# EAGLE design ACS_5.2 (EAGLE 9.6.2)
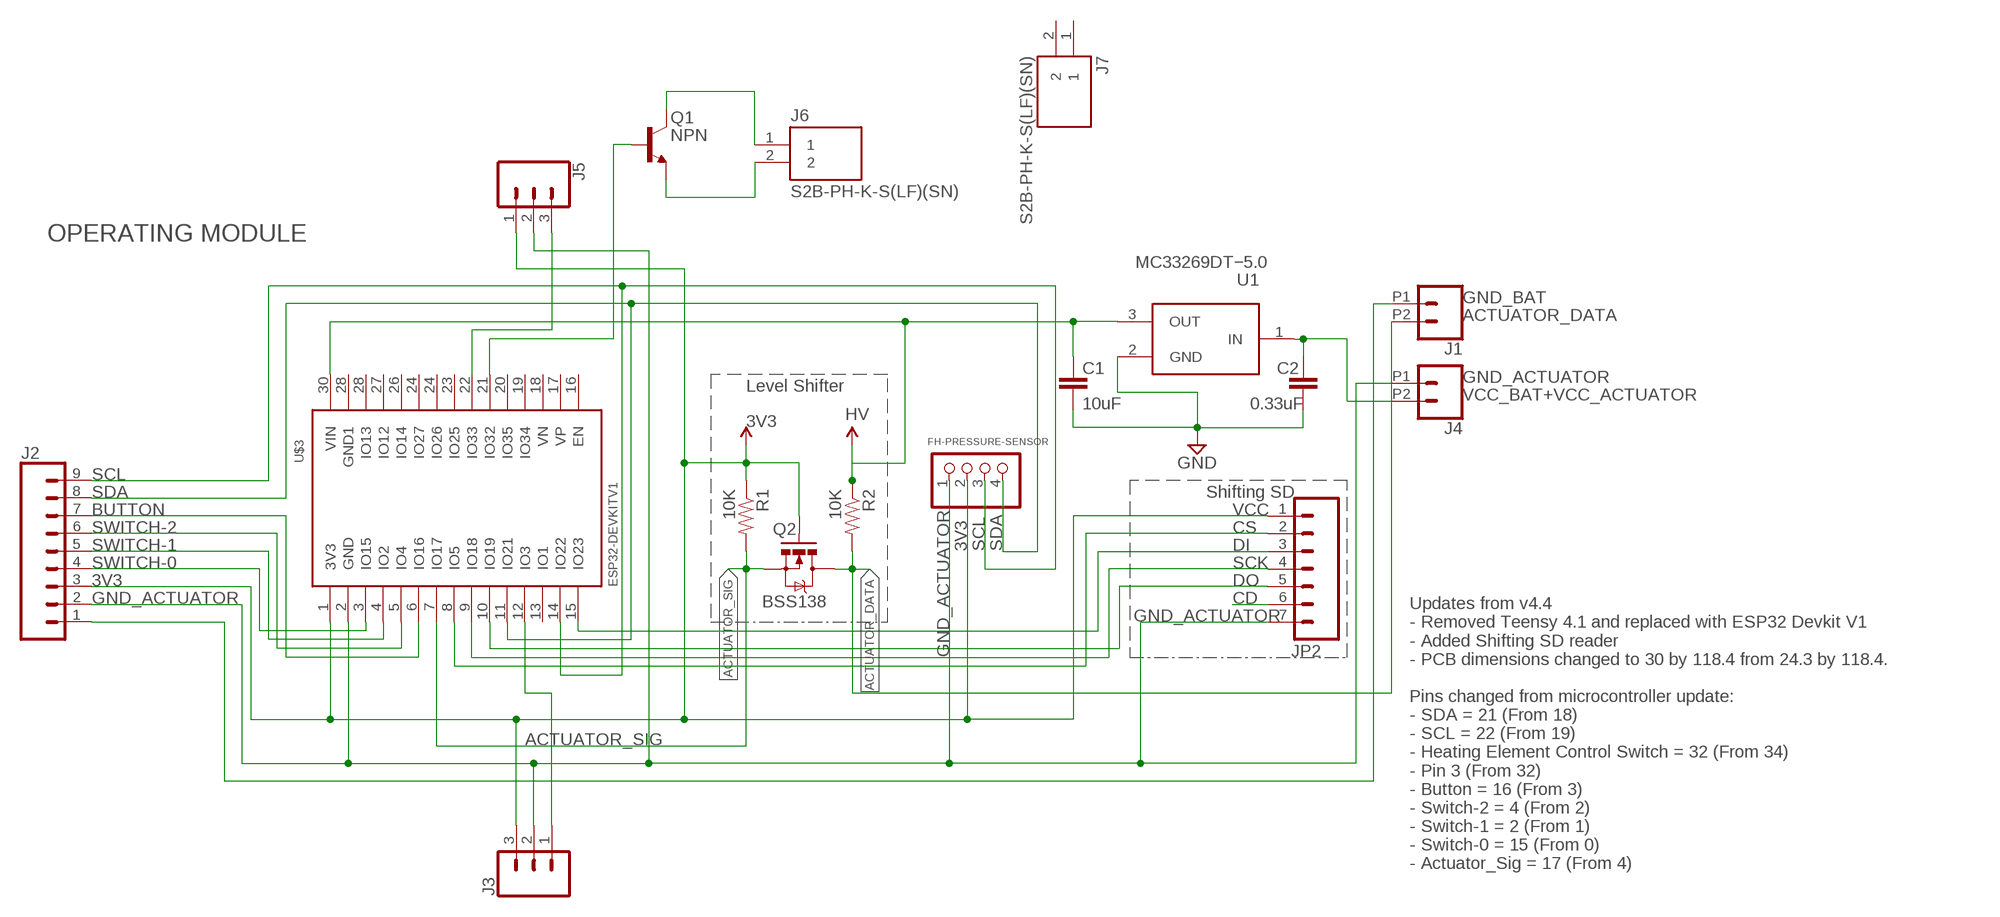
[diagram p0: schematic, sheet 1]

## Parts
C1  10uF  C_CHIP-0603(1608-METRIC)  [CAPC1608X85]
C2  0.33uF  C_CHIP-0603(1608-METRIC)  [CAPC1608X85]
FH-PRESSURE-SENSOR  PINHD-1X4  [1X04]
J1  CONN_022.54MM_SCREWTERM  [1X02_2.54_SCREWTERM]
J2  CONN_09  [1X09]
J3  CONN_03  [1X03]
J4  CONN_022.54MM_SCREWTERM  [1X02_2.54_SCREWTERM]
J5  CONN_03  [1X03]
J6  S2B-PH-K-S(LF)(SN)  [JST_S2B-PH-K-S(LF)(SN)]
J7  S2B-PH-K-S(LF)(SN)  [JST_S2B-PH-K-S(LF)(SN)]
JP2  M07  [1X07]
Q1  NPN  NPN_SOT23  [SOT95P237X112-3N]
Q2  BSS138  MOSFET-NCHANNELSMD  [SOT23-3]
R1  10K  RESISTOR0603-RES  [0603-RES]
R2  10K  RESISTOR0603-RES  [0603-RES]
U1  MC78M05BDTRKG  [MC78M05BDTRKG]
U$3  ESP32DEVKITV1  [ESP32-DEVKITV1]

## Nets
3V3: FH-PRESSURE-SENSOR.2 J2.3 J3.3 J5.1 JP2.1 Q2.1(G) R1.1 U$3.1(3V3) ; supply symbol labelled LV
ACTUATOR_DATA: J1.P2 Q2.3(D) R2.2
ACTUATOR_SIG: Q2.2(S) R1.2 U$3.7(IO17)
BUTTON: J2.7 U$3.6(IO16)
GND: C1.2 C2.2 U1.2(GND)
GND_ACTUATOR: FH-PRESSURE-SENSOR.1 J2.2 J3.2 J4.P1 J5.2 JP2.7 U$3.2(GND)
GND_BAT: J1.P1 J2.1
HV: C1.1 R2.1 U1.3(OUT) U$3.30(VIN)
N$1: J5.3 U$3.22(IO33)
N$3: J6.1 Q1.3(C)
N$4: J6.2 Q1.1(E)
N$5: Q1.2(B) U$3.21(IO32)
N$8: JP2.6
N$10: J3.1 U$3.12(IO3)
N$11: JP2.3 U$3.15(IO23)
N$12: JP2.2 U$3.8(IO5)
N$13: JP2.4 U$3.9(IO18)
N$14: JP2.5 U$3.10(IO19)
SCL: FH-PRESSURE-SENSOR.3 J2.9 U$3.14(IO22)
SDA: FH-PRESSURE-SENSOR.4 J2.8 U$3.11(IO21)
SWITCH-0: J2.4 U$3.3(IO15)
SWITCH-1: J2.5 U$3.4(IO2)
SWITCH-2: J2.6 U$3.5(IO4)
VCC_BAT+VCC_ACTUATOR: C2.1 J4.P2 U1.1(IN)
Unconnected: J7.1 J7.2 U$3.13(IO1) U$3.16(EN) U$3.17(VP) U$3.18(VN) U$3.19(IO34) U$3.20(IO35) U$3.23(IO25) U$3.24(IO26) U$3.24(IO27) U$3.26(IO14) U$3.27(IO12) U$3.28(GND1) U$3.28(IO13)

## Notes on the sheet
- Heating Element 
  Control Switch
- OPERATING MODULE
- Actuator Voltage: 7.5 MAX
- MC33269DT−5.0
- Level Shifter
- Shifting SD
- VCC
- CS
- DI
- SCK
- DO
- CD
- Updates from v4.4
  - Removed Teensy 4.1 and replaced with ESP32 Devkit V1
  - Added Shifting SD reader
  - PCB dimensions changed to 30 by 118.4 from 24.3 by 118.4.
  
  Pins changed from microcontroller update:
  - SDA = 21 (From 18)
  - SCL = 22 (From 19)
  - Heating Element Control Switch = 32 (From 34)
  - Pin 3 (From 32)
  - Button = 16 (From 3)
  - Switch-2 = 4 (From 2)
  - Switch-1 = 2 (From 1)
  - Switch-0 = 15 (From 0)
  - Actuator_Sig = 17 (From 4)

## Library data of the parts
C1 C2 = Capacitor:C: Capacitor - Generic; CATEGORY: Capacitor
FH-PRESSURE-SENSOR = pinhead:PINHD-1X4: PIN HEADER
J1 J4 = SparkFun-Connectors:CONN_02: Multi connection point. Often used as Generic Header-pin footprint for 0.1 inch spaced/style header connections
J2 = SparkFun-Connectors:CONN_09: Multi connection point. Often used as Generic Header-pin footprint for 0.1 inch spaced/style header connections On any of the 0.1 inch spaced packages, you can populate with these: Break Away Headers - Straight (PRT-00116) Break Away Male Headers - Right Angle (PRT-00553) Female Headers (PRT-00115)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
J3 J5 = SparkFun-Connectors:CONN_03: Multi connection point. Often used as Generic Header-pin footprint for 0.1 inch spaced/style header connections On any of the 0.1 inch spaced packages, you can populate with these: Break Away Headers - Straight (PRT-00116) Break Away Male Headers - Right Angle (PRT-00553) Female Headers (PRT-00115)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
J6 J7 = S2B-PH-K-S_LF__SN_:S2B-PH-K-S(LF)(SN): PH Series 2 Position 2.0 mm Through Hole Side Entry Shrouded Header Check availability; AVAILABILITY: In Stock; DESCRIPTION: Connector Header Through Hole, Right Angle 2 position; MF: JST Sales America Inc.; MP: S2B-PH-K-S(LF)(SN); PACKAGE: None; PRICE: None; PURCHASE-URL: https://pricing.snapeda.com/search/part/S2B-PH-K-S(LF)(SN)/?ref=eda
JP2 = SparkFun-Connectors:M07: Header 7 Standard 7-pin 0.1" header. Use with straight break away headers (SKU : PRT-00116), right angle break away headers (PRT-00553), swiss pins (PRT-00743), machine pins (PRT-00117), and female headers (PRT-00115). NOTES ON THE VARIANTS LOCK and LOCK_LONGPADS... This footprint was designed to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
Q1 = Transistor:NPN: NPN - Generic; CATEGORY: Transistor; SUB-CATEGORY: BJT; TYPE: NPN
Q2 = SparkFun:MOSFET-NCHANNEL
R1 R2 = SparkFun:RESISTOR: Resistor
U1 = LDO:MC78M05BDTRKG: IC REG LINEAR 5V 500MA DPAK Manufacturer's datasheet; CREATED_BY: PCBLayout.com; DIGIKEY_PN: MC78M05BDTRKGOSCT-ND; MANUFACTURER: ON Semiconductor; MPN: IC REG LINEAR 5V 500MA DPAK; PACKAGE: DPak
U$3 = ESP32-DEVKITV1:ESP32DEVKITV1

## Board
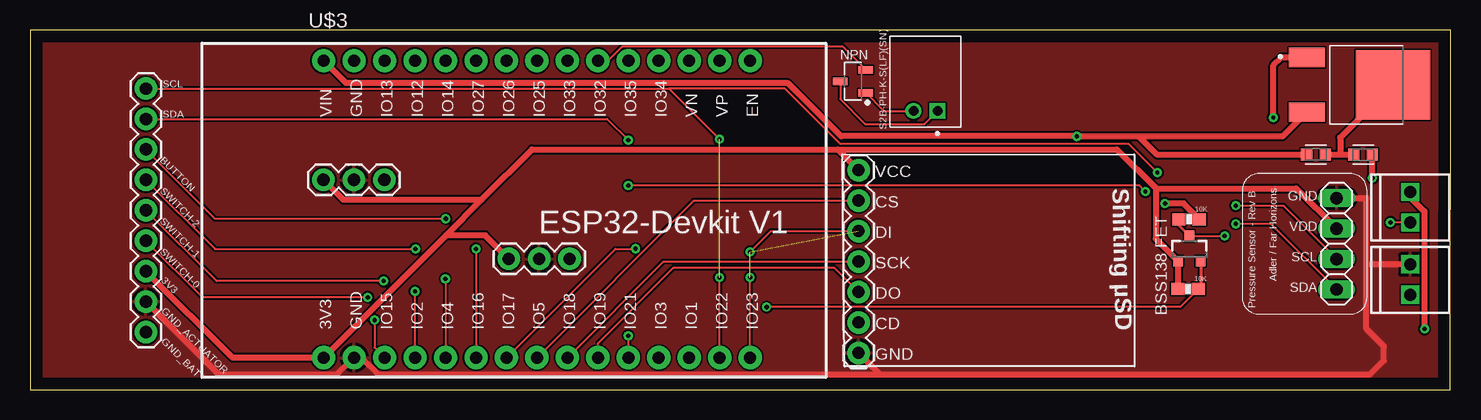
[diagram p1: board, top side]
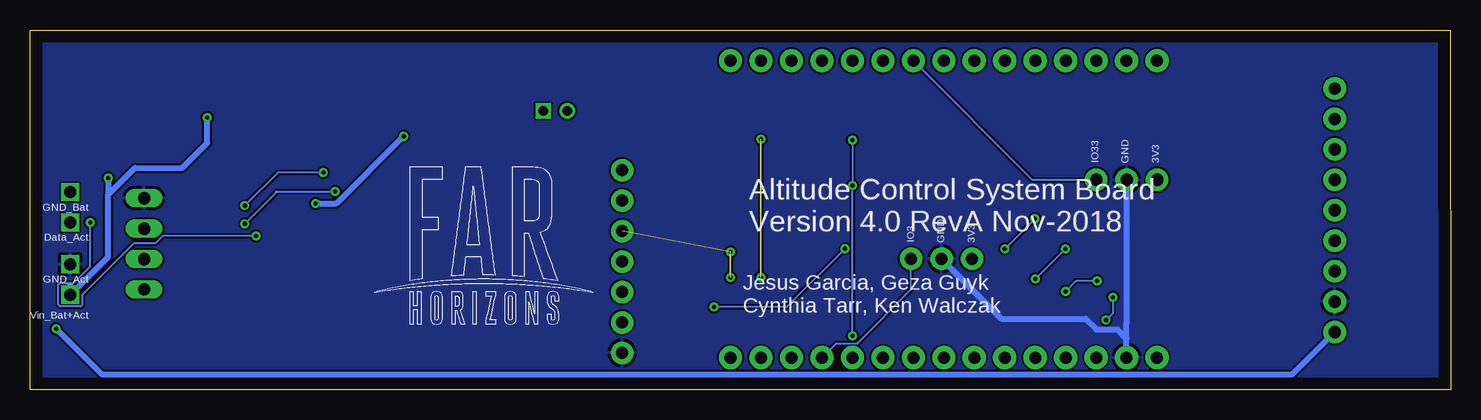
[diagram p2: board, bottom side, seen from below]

Size 118.43 x 30 mm. Coordinates in mm from the lower left corner, seen from the top.
Outline: 0,0 118.4,0 118.43,30 0.03,30 0,0
Copper layers (1*16): Top 0.035mm / dielectric 1.5mm / Bottom 0.035mm
Design rules "default": minimum track width 6mil, minimum drill 0.35mm, track to track 6mil, track to pad 6mil, pad to pad 6mil, via to via 6mil, smd to smd 6mil, copper to edge 40mil, drill to drill 6mil, minimum pad ring 10mil, minimum via ring 8mil, stop-mask expansion 4mil, vias tented up to drill 0mil, thermal gap 10mil

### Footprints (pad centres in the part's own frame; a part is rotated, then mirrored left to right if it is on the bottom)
CAPC1608X85 = smd 0.921 x 0.97: 1 -0.775,0; 2 0.775,0
1X04 = drill 1.016 long: 1 -3.81,0; 2 -1.27,0; 3 1.27,0; 4 3.81,0
1X02_2.54_SCREWTERM = drill 1.016 square: P1 2.54,0; P2 0,0
1X09 = drill 1.016 pad 1.88: 1 0,0; 2 2.54,0; 3 5.08,0; 4 7.62,0; 5 10.16,0; 6 12.7,0; 7 15.24,0; 8 17.78,0; 9 20.32,0
1X03 = drill 1.016 pad 1.88: 1 0,0; 2 2.54,0; 3 5.08,0
JST_S2B-PH-K-S(LF)(SN) = drill 0.8 square: 1 -1,0 | drill 0.8: 2 1,0
1X07 = drill 1.016 pad 1.88: 1 0,0; 2 2.54,0; 3 5.08,0; 4 7.62,0; 5 10.16,0; 6 12.7,0; 7 15.24,0
SOT95P237X112-3N = smd 1.224 x 0.625: 1 -1.064,0.95; 2 -1.064,-0.95; 3 1.064,0
SOT23-3 = smd 0.8 x 0.9: 1 -0.95,-1; 2 0.95,-1; 3 0,1.1
0603-RES = smd 1.1 x 1: 1 -0.85,0; 2 0.85,0
MC78M05BDTRKG = smd 1.6 x 3: 1 -2.285,-4.08; 3 2.285,-4.08 | smd 5.8 x 6.2: 2 0,3.1
ESP32-DEVKITV1 = drill 1 pad 1.93: 1 -22.87,-13.54; 2 -20.33,-13.54; 3 -17.79,-13.54; 4 -15.25,-13.54; 5 -12.71,-13.54; 6 -10.17,-13.54; 7 -7.63,-13.54; 8 -5.09,-13.54; 9 -2.55,-13.54; 10 -0.01,-13.54; 11 2.53,-13.54; 12 5.07,-13.54; 13 7.61,-13.54; 14 10.15,-13.54; 15 12.69,-13.54; 16 12.69,11.23; 17 10.15,11.23; 18 7.61,11.23; 19 5.07,11.23; 20 2.53,11.23; 21 -0.01,11.23; 22 -2.55,11.23; 23 -5.09,11.23; 24 -7.63,11.23; 25 -10.17,11.23; 26 -12.71,11.23; 27 -15.25,11.23; 28 -17.79,11.23; 29 -20.33,11.23; 30 -22.87,11.23

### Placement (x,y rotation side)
C1  107.19,19.61 0 top
C2  111.13,19.6 180 top
FH-PRESSURE-SENSOR  108.92,12.15 270 top
J1  115.07,13.94 90 top
J2  9.66,4.79 90 top
J3  44.98,10.9 180 top
J4  115.07,7.91 90 top
J5  24.46,17.5 0 top
J6  74.65,23.25 180 top
J7  not placed on the board
JP2  69.07,18.3 270 top
Q1  68.61,25.72 180 top
Q2  96.65,11.72 0 top
R1  96.56,8.41 0 top
R2  96.62,14.21 180 top
U1  110.51,25.42 270 top
U$3  47.34,16.2 0 top

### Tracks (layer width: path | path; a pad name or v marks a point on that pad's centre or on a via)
3V3
  Top 0.152: 95.7,8.42 R1.1
  Top 0.254: 95.68,10.73 Q2.1
  Top 0.508: J2.3 16.88,2.65 U$3.1 34.67,12.86 | 34.67,12.86 37.66,15.85 | 37.66,15.85 41.84,20.03 67.34,20.03 | JP2.1 67.34,20.03 | 67.34,20.03 90.6,20.03 93.84,16.79 93.84,16.78 | 93.84,16.78 105.56,16.78 FH-PRESSURE-SENSOR.2 | 93.84,16.78 93.84,12.57 Q2.1 95.69,10.71 95.69,8.42 R1.1 | J5.1 26.11,15.85 37.66,15.85 | J3.3 37.94,12.86 34.67,12.86
ACTUATOR_DATA  (via drill 0.35)
  Top 0.152: Q2.3 v99.59,12.82 | J1.P2 v113.41,13.94
  Top 0.254: R2.2 95.77,13.7 Q2.3
  Bottom 0.152: v99.59,12.82 107.36,12.82 107.98,12.2 109.76,12.2 114.08,7.89 114.08,7.05 114.21,6.92 115.93,6.92 116.06,7.05 116.06,8.76 115.93,8.9 114.77,8.9 113.41,10.26 v113.41,13.94
ACTUATOR_SIG  (via drill 0.35)
  Top 0.152: 97.47,8.48 R1.2 95.88,6.88 v61.41,6.88 | U$3.7 48.8,11.75 v50.48,11.75
  Top 0.254: Q2.2 97.6,8.6 97.47,8.48
  Bottom 0.152: v50.48,11.75 55.35,6.88 v61.41,6.88
BUTTON  (via drill 0.35)
  Top 0.152: v37.17,11.74 U$3.6 | v34.66,14.25 15.44,14.25 J2.7
  Bottom 0.152: v34.66,14.25 v37.17,11.74
GND
  Top 0.508: C1.2 109.22,19.61 | 109.22,19.61 110.34,19.61 C2.2 | 109.22,19.61 109.22,21.03 U1.2
GND_ACTUATOR
  Top 0.508: J2.2 15.73,1.27 25.62,1.27 U$3.2 27.61,2.67 29.01,1.27 70.86,1.27 | 70.86,1.27 111.7,1.27 112.86,2.43 112.86,3.6 111.4,5.06 111.4,10.61 | JP2.7 70.86,1.27 | J4.P1 111.56,10.45 111.4,10.61 | 111.4,10.61 111.4,15.95 111.39,15.96 FH-PRESSURE-SENSOR.1
  Bottom 0.508: U$3.2 27.02,4.25 | 27.02,4.25 27.02,5.51 27,5.53 J5.2 | J3.2 37.43,5.9 30.44,5.9 29.55,5.01 27.77,5.01 27.02,4.25
  pour Top: -4.15,31.64 -4.15,-1.81 119.4,-1.81 119.4,31.64
  pour Bottom: -5.76,31.6 -5.76,-1.75 119.61,-1.75 119.61,31.6
GND_BAT  (via drill 0.35)
  Top 0.508: J1.P1 115.07,16.04 116.25,14.86 v116.25,5.07 v116.25,5.06
  Bottom 0.508: v116.25,5.06 112.46,1.27 13.18,1.27 J2.1
HV  (via drill 0.35)
  Top 0.508: 24.48,27.43 26.31,25.6 63.13,25.6 67.61,21.13 v87.27,21.13 92.41,21.13 | 24.48,27.43 | U$3.30 24.48,27.43 | R2.1 96.15,15.52 v94.62,15.52 | 92.41,21.13 93.93,19.61 C1.1 | 92.41,21.13 104.42,21.13 U1.3
  Bottom 0.508: v94.62,15.52 92.88,15.52 v87.27,21.13
N$1
  Bottom 0.152: J5.3 34.86,17.5 U$3.22
N$3
  Top 0.152: Q1.3 67.55,24.23 69.62,22.16 74.56,22.16 J6.1
N$4
  Top 0.152: Q1.1 71.19,23.25 J6.2
N$5
  Top 0.152: U$3.21 48.19,27.43 49.38,28.63 61.13,28.63 61.22,28.63 67.72,28.63 Q1.2
N$10
  Bottom 0.152: U$3.12 51.22,3.86 49.46,3.86 44.98,8.35 J3.1
N$11  (via drill 0.35)  (2 unrouted)
  Top 0.152: U$3.15 v60.03,9.35 | v60.03,11.48 61.77,13.22 JP2.3
  Bottom 0.152: v60.03,9.35 v60.03,11.48
N$12
  Top 0.152: U$3.8 55.35,15.76 JP2.2
N$13
  Top 0.152: U$3.9 52.81,10.68 JP2.4
N$14
  Top 0.152: U$3.10 47.34,3.85 53.61,10.13 67.08,10.13 JP2.5
SCL  (via drill 0.35)  (3 unrouted)
  Top 0.152: U$3.14 v57.49,9.35 v57.49,9.36 | J2.9 53.25,25.11 | 53.25,25.11 v57.49,20.88 | v93.98,18.11 91.56,20.52 67.53,20.52 62.94,25.11 53.25,25.11 | v100.52,15.34 104.46,15.34 FH-PRESSURE-SENSOR.3
  Bottom 0.152: v57.49,9.36 v57.49,20.88 | v93.98,18.11 97.75,18.11 v100.52,15.34
SDA  (via drill 0.35)
  Top 0.152: J2.8 48.12,22.57 | v92.98,16.53 92.48,17.03 v49.88,17.03 | FH-PRESSURE-SENSOR.4 103.43,13.83 v100.52,13.83 | v49.88,20.82 48.12,22.57 | 48.12,22.57 | U$3.11 v49.88,4.49
  Bottom 0.152: v100.52,13.83 97.91,16.44 97.91,16.53 v92.99,16.53 v92.98,16.53 | v49.88,20.82 v49.88,17.03 v49.88,4.49
SWITCH-0  (via drill 0.35)
  Top 0.152: v28.16,7.7 14.38,7.7 J2.4 | v28.73,5.8 28.71,5.79 28.71,3.5 U$3.3
  Bottom 0.152: v28.73,5.8 28.18,6.34 28.18,7.68 v28.16,7.7
SWITCH-1  (via drill 0.35)
  Top 0.152: v29.47,9.06 15.55,9.06 J2.5 | U$3.4 v32.09,8.19
  Bottom 0.152: v29.47,9.06 31.23,9.06 v32.09,8.19
SWITCH-2  (via drill 0.35)
  Top 0.152: v34.62,9.23 34.62,2.67 U$3.5 | J2.6 15.43,11.72 v32.13,11.72
  Bottom 0.152: v34.62,9.23 v32.13,11.72
VCC_BAT+VCC_ACTUATOR  (via drill 0.35)
  Top 0.508: v111.91,17.65 C2.1 | U1.1 104.3,27.7 103.65,27.06 v103.65,22.68
  Bottom 0.508: J4.P2 111.91,11.07 111.91,16.27 | v111.91,17.65 111.91,16.27 | 111.91,16.27 109.69,18.49 105.74,18.49 103.65,20.58 v103.65,22.68

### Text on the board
tPlace: Shifting µSD
bPlace: Altitude Control System Board / Version 4.0 RevA Nov-2018 | Jesus Garcia, Geza Guyk / Cynthia Tarr, Ken Walczak
tNames: NPN | SCL | SDA | S2B-PH-K-S(LF)(SN) | BUTTON | VCC | SWITCH-2 | Pressure Sensor - Rev B | Adler / Far Horizons | GND | CS | 10K | SWITCH-1 | VDD | DI | SWITCH-0 | SCL | SCK | 3V3 | 10K | SDA | DO | GND_ACTUATOR | BSS138 FET | CD | GND_BAT | GND
bNames: GND | IO33 | 3V3 | GND_Bat | 3V3 | GND | IO3 | Data_Act | GND_Act | Vin_Bat+Act
tValues: 10uF | 0.33uF

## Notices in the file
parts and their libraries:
SparkFun-Connectors: Licensing: Creative Commons ShareAlike 4.0 International - https://creativecommons.org/licenses/by-sa/4.0
SparkFun-Connectors: Licensing: CC v3.0 Share-Alike You are welcome to use this library for commercial purposes.
